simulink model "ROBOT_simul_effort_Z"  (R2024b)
settings: Solver=VariableStepAuto  StartTime=0.0  StopTime=5  RelTol=1e-3
undefined symbols (not defined in the file): a, ARRIERE_Defaut_sldprt, avant01_Defaut_sldprt, avant02_Defaut_sldprt, avant03_Defaut_sldprt, avant1_Defaut_sldprt, AXE, BASE_Defaut_sldprt, BIELLE, BIELLE_Defaut_sldprt, BRAS_Defaut_sldprt, bras_Defaut_sldprt, C_Realiste_sldprt, CABLE_Defaut_sldprt, cable_Defaut_sldprt, CACHE_Defaut_sldprt, CARTE, carte_Defaut_sldprt, CARTER, carter, CHC, CODEUR_Defaut_sldprt, cruciforme, cylindrique, deg, Drive, Fichiers, Fichiers_Matlab_sujetA, FIXATION, fixation_Defaut_sldprt, H, HEXAGONALE_Defaut_sldprt, joint_Defaut_sldprt, kg, m, M4, M4_Defaut_sldprt, manette1_Defaut_sldprt, manette2_Defaut_sldprt, MATLAB, Matlab, matlab_Defaut_sldprt, mm, modif, MOTEUR_Defaut_sldprt, N, NEZ_Defaut_sldprt, nom, palier, PARALLELOGRAMME_Defaut_sldprt, petite, plaque, rad, Ressort, Rondelle, ROTOR_Defaut_sldprt, s, SET, simple, socle_Defaut_sldprt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
libraries: sm_lib x463, fl_lib x45, nesl_utility x27, simulink x2
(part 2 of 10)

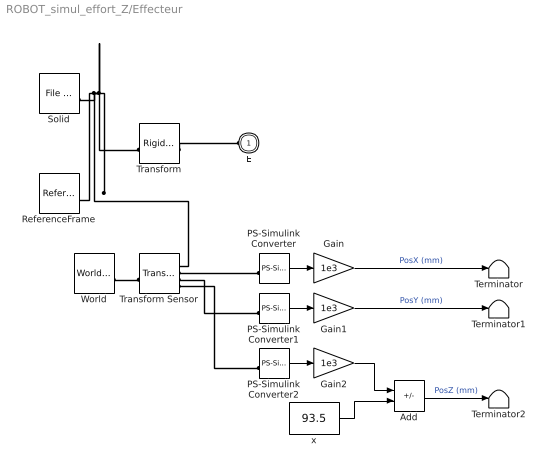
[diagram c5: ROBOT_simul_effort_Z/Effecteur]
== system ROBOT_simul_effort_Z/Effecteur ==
  Add : Sum  Inputs=+-
  Gain : Gain  Gain=1e3
  Gain1 : Gain  Gain=1e3
  Gain2 : Gain  Gain=1e3
  PS-Simulink Converter : nesl_utility/PS-Simulink Converter  PhysicalDomain=network_engine_domain  SubClassName=ps_output  LeftPortType=input  RightPortType=output  PseudoPeriodic=off  Frequencies=[]  VectorFormat=1-D array  Unit=1  AffineConversion=off
  PS-Simulink Converter1 : nesl_utility/PS-Simulink Converter  PhysicalDomain=network_engine_domain  SubClassName=ps_output  LeftPortType=input  RightPortType=output  PseudoPeriodic=off  Frequencies=[]  VectorFormat=1-D array  Unit=1  AffineConversion=off
  PS-Simulink Converter2 : nesl_utility/PS-Simulink Converter  PhysicalDomain=network_engine_domain  SubClassName=ps_output  LeftPortType=input  RightPortType=output  PseudoPeriodic=off  Frequencies=[]  VectorFormat=1-D array  Unit=1  AffineConversion=off
  ReferenceFrame : sm_lib/Frames and Transforms/Reference Frame
  Solid : sm_lib/Body Elements/File Solid  ExtGeomFileName=/MATLAB Drive/Fichiers_Matlab_sujetA/Fichiers Matlab/STL/manette2_Defaut_sldprt.STL  UnitType=Custom  ExtGeomFileUnits=mm  StepReaderType=HEX  ExportConvexHullGeometry=off  InertiaType=Custom  BasedOnType=Density  Density=1000  DensityUnits=kg/(m^3)  Mass=0.053  MassUnits=kg  CenterOfMass=[0 0 35.7]  CenterOfMassUnits=mm  MomentsOfInertia=[11.53195593564609 11.464562757624146 11.477456236480506]  MomentsOfInertiaUnits=kg*mm^2  ProductsOfInertia=[-0.014032469477280249 0.0038968914795150661 0.025527028661124163]  ProductsOfInertiaUnits=kg*mm^2  GraphicType=FromGeometry  MarkerShape=Sphere  MarkerSize=10  GraphicVisPropType=SimpleVisualProperties  GraphicDiffuseColor=[1 1 1]  GraphicOpacity=1  GraphicSpecularColor=[0.5 0.5 0.5 1.0]  GraphicAmbientColor=[0.15 0.15 0.15 1.0]  GraphicEmissiveColor=[0.0 0.0 0.0 1.0]  GraphicShininess=75  DoExposeReferenceFrame=on  SerializedFrames=<Frames/>
  Terminator : Terminator
  Terminator1 : Terminator
  Terminator2 : Terminator
  Transform : sm_lib/Frames and Transforms/Rigid Transform  RotationMethod=ArbitraryAxis  FollAlignAxisA=+X  BaseAlignAxisA=+Y  FollAlignAxisB=+Y  BaseAlignAxisB=+Z  RotationStandardAxis=+Z  RotationAngle=2.2920311904365782  RotationAngleUnits=rad  RotationArbitraryAxis=[0.63063758405056181 -0.45231899713116352 0.63063758405056158]  RotationSequenceAxes=FollowerAxes  RotationSequence=XYX  RotationSequenceAngles=[0 0 0]  RotationSequenceAnglesUnits=deg  RotationMatrix=[1 0 0; 0 1 0; 0 0 1]  Quaternion=[1 0 0 0]  TranslationMethod=Cartesian  TranslationCartesianOffset=[-0.52204305767083048 1.5422448888264837 -2.2456176397956377e-14]  TranslationCartesianOffsetUnits=mm  TranslationStandardAxis=+Z  TranslationStandardOffset=0  TranslationStandardOffsetUnits=mm  TranslationROffset=0  TranslationROffsetUnits=m  TranslationThetaOffset=0  TranslationThetaOffsetUnits=deg  TranslationZOffset=0  TranslationZOffsetUnits=m
  Transform Sensor : sm_lib/Frames and Transforms/Transform Sensor  MeasurementFrame=World  RotationSequence=XYX  SenseAngle=off  SenseAxis=off  SenseQ=off  SenseR=off  SenseRotationSequence=off  SenseOmegaX=off  SenseOmegaY=off  SenseOmegaZ=off  SenseOmega=off  SenseQDot=off  SenseRDot=off  SenseRotationSequenceDot=off  SenseAlphaX=off  SenseAlphaY=off  SenseAlphaZ=off  SenseAlpha=off  SenseQDDot=off  SenseRDDot=off  SenseX=on  SenseY=on  SenseZ=on  SenseXYZ=off  SenseRad=off  SenseAzim=off  SenseDist=off  SenseInc=off  SenseXDot=off  SenseYDot=off  SenseZDot=off  SenseXYZDot=off  SenseRadDot=off  SenseAzimDot=off  SenseDistDot=off  SenseIncDot=off  SenseXDDot=off  SenseYDDot=off  SenseZDDot=off  SenseXYZDDot=off  SenseRadDDot=off  SenseAzimDDot=off  SenseDistDDot=off  SenseIncDDot=off
  World : sm_lib/Frames and Transforms/World Frame
  x : Constant  Value=93.5
  E : PMIOPort  Side=Left
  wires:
  Gain1/1 -> Terminator1/1  "PosY (mm)"
  PS-Simulink Converter2/1 -> Gain2/1
  x/1 -> Add/2
  Add/1 -> Terminator2/1  "PosZ (mm)"
  PS-Simulink Converter1/1 -> Gain1/1
  Gain2/1 -> Add/1
  PS-Simulink Converter/1 -> Gain/1
  Gain/1 -> Terminator/1  "PosX (mm)"
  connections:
  Solid/RConn1 -- ReferenceFrame/RConn1 -- Transform Sensor/RConn1 -- Transform/LConn1
  Transform/RConn1 -- E/RConn1
  Transform Sensor/RConn3 -- PS-Simulink Converter1/LConn1
  World/RConn1 -- Transform Sensor/LConn1
  PS-Simulink Converter2/LConn1 -- Transform Sensor/RConn4
  Transform Sensor/RConn2 -- PS-Simulink Converter/LConn1

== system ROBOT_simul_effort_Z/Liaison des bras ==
  EFFECTEUR_1_RIGID : Subsystem
  manette_1_RIGID : Subsystem
  E1 : PMIOPort  Side=Left
  E2 : PMIOPort  Port=2  Side=Left
  S1 : PMIOPort  Port=3  Side=Right
  E3 : PMIOPort  Port=4  Side=Left
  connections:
  EFFECTEUR_1_RIGID/RConn1 -- manette_1_RIGID/LConn1
  S1/RConn1 -- manette_1_RIGID/RConn1
  EFFECTEUR_1_RIGID/LConn1 -- E2/RConn1
  EFFECTEUR_1_RIGID/LConn3 -- E1/RConn1
  EFFECTEUR_1_RIGID/LConn2 -- E3/RConn1

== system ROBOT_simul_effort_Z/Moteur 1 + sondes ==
  In1 : Inport
  Moteur courant continu1 : Subsystem
  Reference electrique : fl_lib/Electrical/Electrical Elements/Electrical Reference
  Simulink-PS Converter1 : nesl_utility/Simulink-PS Converter  PhysicalDomain=network_engine_domain  SubClassName=ps_input  LeftPortType=input  RightPortType=output  PseudoPeriodic=off  Frequencies=[]  NoiseDistribution=none  NoiseParameters=[]  Unit=V  AffineConversion=off  FilteringAndDerivatives=zero  SimscapeFilterOrder=2  InputFilterTimeConstant=1e-4  UdotUserProvided=1
  Sondes electriques1 : Subsystem
  Source de tension controlée1 : fl_lib/Electrical/Electrical Sources/Controlled Voltage Source
  Conn1 : PMIOPort  Side=Right
  Conn2 : PMIOPort  Port=2  Side=Right
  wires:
  In1/1 -> Simulink-PS Converter1/1
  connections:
  Conn2/RConn1 -- Moteur courant continu1/RConn2
  Conn1/RConn1 -- Moteur courant continu1/RConn1
  Source de tension controlée1/LConn1 -- Sondes electriques1/LConn1
  Simulink-PS Converter1/RConn1 -- Source de tension controlée1/RConn1
  Sondes electriques1/RConn2 -- Source de tension controlée1/RConn2 -- Reference electrique/LConn1 -- Moteur courant continu1/LConn2
  Sondes electriques1/RConn1 -- Moteur courant continu1/LConn1

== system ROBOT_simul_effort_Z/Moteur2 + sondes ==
  In1 : Inport
  Moteur courant continu2 : Subsystem
  Reference electrique : fl_lib/Electrical/Electrical Elements/Electrical Reference
  Simulink-PS Converter1 : nesl_utility/Simulink-PS Converter  PhysicalDomain=network_engine_domain  SubClassName=ps_input  LeftPortType=input  RightPortType=output  PseudoPeriodic=off  Frequencies=[]  NoiseDistribution=none  NoiseParameters=[]  Unit=V  AffineConversion=off  FilteringAndDerivatives=zero  SimscapeFilterOrder=2  InputFilterTimeConstant=1e-4  UdotUserProvided=1
  Sondes electriques : Subsystem
  Source de tension controlée : fl_lib/Electrical/Electrical Sources/Controlled Voltage Source
  Conn1 : PMIOPort  Side=Right
  Conn2 : PMIOPort  Port=2  Side=Right
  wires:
  In1/1 -> Simulink-PS Converter1/1
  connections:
  Sondes electriques/RConn1 -- Moteur courant continu2/LConn1
  Source de tension controlée/RConn2 -- Reference electrique/LConn1 -- Sondes electriques/RConn2 -- Moteur courant continu2/LConn2
  Simulink-PS Converter1/RConn1 -- Source de tension controlée/RConn1
  Source de tension controlée/LConn1 -- Sondes electriques/LConn1
  Conn1/RConn1 -- Moteur courant continu2/RConn1
  Conn2/RConn1 -- Moteur courant continu2/RConn2

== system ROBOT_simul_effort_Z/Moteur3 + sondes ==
  In1 : Inport
  Moteur courant continu3 : Subsystem
  Reference electrique : fl_lib/Electrical/Electrical Elements/Electrical Reference
  Simulink-PS Converter1 : nesl_utility/Simulink-PS Converter  PhysicalDomain=network_engine_domain  SubClassName=ps_input  LeftPortType=input  RightPortType=output  PseudoPeriodic=off  Frequencies=[]  NoiseDistribution=none  NoiseParameters=[]  Unit=V  AffineConversion=off  FilteringAndDerivatives=zero  SimscapeFilterOrder=2  InputFilterTimeConstant=1e-4  UdotUserProvided=1
  Sondes electriques3 : Subsystem
  Source de tension controlée3 : fl_lib/Electrical/Electrical Sources/Controlled Voltage Source
  Conn1 : PMIOPort  Side=Right
  Conn2 : PMIOPort  Port=2  Side=Right
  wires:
  In1/1 -> Simulink-PS Converter1/1
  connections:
  Sondes electriques3/RConn1 -- Moteur courant continu3/LConn1
  Moteur courant continu3/LConn2 -- Reference electrique/LConn1 -- Source de tension controlée3/RConn2 -- Sondes electriques3/RConn2
  Simulink-PS Converter1/RConn1 -- Source de tension controlée3/RConn1
  Source de tension controlée3/LConn1 -- Sondes electriques3/LConn1
  Conn1/RConn1 -- Moteur courant continu3/RConn1
  Conn2/RConn1 -- Moteur courant continu3/RConn2

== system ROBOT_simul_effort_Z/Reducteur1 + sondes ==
  Conv en tr/s : Gain  Gain=-60/(2*pi)
  Conv w : nesl_utility/PS-Simulink Converter  PhysicalDomain=network_engine_domain  SubClassName=ps_output  LeftPortType=input  RightPortType=output  PseudoPeriodic=off  Frequencies=[]  VectorFormat=1-D array  Unit=1  AffineConversion=off
  Conv w1 : nesl_utility/PS-Simulink Converter  PhysicalDomain=network_engine_domain  SubClassName=ps_output  LeftPortType=input  RightPortType=output  PseudoPeriodic=off  Frequencies=[]  VectorFormat=1-D array  Unit=1  AffineConversion=off
  Invers signe : Gain  Gain=-1
  Reference mecanique : fl_lib/Mechanical/Rotational Elements/Mechanical Rotational Reference
  Rotational Hard Stop : fl_lib/Mechanical/Rotational Elements/Rotational Hard Stop  Commented=on  upper_bnd=0 rad  lower_bnd=-1.95 rad  model=simscape.enum.hardstop.fulldamped  stiff_up=1e+4 N*m/rad  stiff_low=1e+4 N*m/rad  D_up=100 N*m/(rad/s)  D_low=100 N*m/(rad/s)  transition=0.001 rad  coeff_rest=0.7  w_tol=0.1 rad/s  trq_tol=0.001 N*m  w_specify=off  w_priority=None  w=0 rad/s  w_nominal_specify=off  w_nominal_value=1  w_nominal_unit=rad/s  t_specify=off  t_priority=None  t=0 N*m  t_nominal_specify=off  t_nominal_value=1  t_nominal_unit=N*m  phi_specify=on  phi_priority=High  phi=0 rad  phi_nominal_specify=off  phi_nominal_value=1  phi_nominal_unit=rad  M_specify=off  M_priority=None  M=0
  Réducteur de vitesse : fl_lib/Mechanical/Mechanisms/Gear Box  ratio=-7.627  t_in_specify=off  t_in_priority=None  t_in=0 N*m  t_in_nominal_specify=off  t_in_nominal_value=1  t_in_nominal_unit=N*m  t_out_specify=off  t_out_priority=None  t_out=0 N*m  t_out_nominal_specify=off  t_out_nominal_value=1  t_out_nominal_unit=N*m
  Sonde omega /theta1 : fl_lib/Mechanical/Mechanical Sensors/Ideal Rotational Motion Sensor  reference=foundation.enum.MeasurementReference.difference  acceleration_port=false  velocity_port=true  position_port=true  wrap_angle=false  offset=0 rad
  Terminator : Terminator
  Terminator1 : Terminator
  E1 : PMIOPort  Side=Left
  Ref : PMIOPort  Port=2  Side=Left
  S1 : PMIOPort  Port=3  Side=Right
  Ref1 : PMIOPort  Port=4  Side=Right
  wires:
  Conv w1/1 -> Invers signe/1  "Angle_mot1 (rad)"
  Invers signe/1 -> Terminator1/1  "Angle_mot1 (rad)"
  Conv w/1 -> Conv en tr/s/1
  Conv en tr/s/1 -> Terminator/1  "Nmoteur1 (tr/min)"
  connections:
  Sonde omega /theta1/LConn1 -- E1/RConn1 -- Réducteur de vitesse/LConn1
  Reference mecanique/LConn1 -- Ref/RConn1 -- Ref1/RConn1 -- Rotational Hard Stop/RConn1 -- Sonde omega /theta1/RConn1
  Conv w/LConn1 -- Sonde omega /theta1/RConn2
  Conv w1/LConn1 -- Sonde omega /theta1/RConn3
  Réducteur de vitesse/RConn1 -- Rotational Hard Stop/LConn1 -- S1/RConn1

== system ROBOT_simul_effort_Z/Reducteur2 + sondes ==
  Conv en tr/s : Gain  Gain=60/(2*pi)
  Conv en ° : Gain  Gain=180/pi
  Conv w : nesl_utility/PS-Simulink Converter  PhysicalDomain=network_engine_domain  SubClassName=ps_output  LeftPortType=input  RightPortType=output  PseudoPeriodic=off  Frequencies=[]  VectorFormat=1-D array  Unit=1  AffineConversion=off
  Conv w1 : nesl_utility/PS-Simulink Converter  PhysicalDomain=network_engine_domain  SubClassName=ps_output  LeftPortType=input  RightPortType=output  PseudoPeriodic=off  Frequencies=[]  VectorFormat=1-D array  Unit=1  AffineConversion=off
  Reference mecanique : fl_lib/Mechanical/Rotational Elements/Mechanical Rotational Reference
  Rotational Hard Stop : fl_lib/Mechanical/Rotational Elements/Rotational Hard Stop  Commented=on  upper_bnd=1.95 rad  lower_bnd=0 rad  model=simscape.enum.hardstop.fulldamped  stiff_up=1e+4 N*m/rad  stiff_low=1e+4 N*m/rad  D_up=100 N*m/(rad/s)  D_low=100 N*m/(rad/s)  transition=0.001 rad  coeff_rest=0.7  w_tol=0.1 rad/s  trq_tol=0.001 N*m  w_specify=off  w_priority=None  w=0 rad/s  w_nominal_specify=off  w_nominal_value=1  w_nominal_unit=rad/s  t_specify=off  t_priority=None  t=0 N*m  t_nominal_specify=off  t_nominal_value=1  t_nominal_unit=N*m  phi_specify=on  phi_priority=High  phi=0 rad  phi_nominal_specify=off  phi_nominal_value=1  phi_nominal_unit=rad  M_specify=off  M_priority=None  M=0
  Réducteur de vitesse2 : fl_lib/Mechanical/Mechanisms/Gear Box  ratio=7.627  t_in_specify=off  t_in_priority=None  t_in=0 N*m  t_in_nominal_specify=off  t_in_nominal_value=1  t_in_nominal_unit=N*m  t_out_specify=off  t_out_priority=None  t_out=0 N*m  t_out_nominal_specify=off  t_out_nominal_value=1  t_out_nominal_unit=N*m
  Sonde omega /theta2 : fl_lib/Mechanical/Mechanical Sensors/Ideal Rotational Motion Sensor  reference=foundation.enum.MeasurementReference.difference  acceleration_port=false  velocity_port=true  position_port=true  wrap_angle=false  offset=0 rad
  Terminator : Terminator
  Terminator1 : Terminator
  E1 : PMIOPort  Side=Left
  Ref : PMIOPort  Port=2  Side=Left
  S1 : PMIOPort  Port=3  Side=Right
  Ref1 : PMIOPort  Port=4  Side=Right
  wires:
  Conv w1/1 -> Conv en °/1  "Angle_mot2 (rad)"
  Conv en °/1 -> Terminator1/1  "Angle_mot2 (°)"
  Conv w/1 -> Conv en tr/s/1
  Conv en tr/s/1 -> Terminator/1  "Nmoteur2 (tr/min)"
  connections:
  Sonde omega /theta2/LConn1 -- E1/RConn1 -- Réducteur de vitesse2/LConn1
  Ref1/RConn1 -- Sonde omega /theta2/RConn1 -- Reference mecanique/LConn1 -- Ref/RConn1 -- Rotational Hard Stop/RConn1
  Conv w1/LConn1 -- Sonde omega /theta2/RConn3
  Conv w/LConn1 -- Sonde omega /theta2/RConn2
  Réducteur de vitesse2/RConn1 -- Rotational Hard Stop/LConn1 -- S1/RConn1

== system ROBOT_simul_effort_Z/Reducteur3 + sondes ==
  Conv en tr/s : Gain  Gain=60/(2*pi)
  Conv en ° : Gain  Gain=180/pi
  Conv w : nesl_utility/PS-Simulink Converter  PhysicalDomain=network_engine_domain  SubClassName=ps_output  LeftPortType=input  RightPortType=output  PseudoPeriodic=off  Frequencies=[]  VectorFormat=1-D array  Unit=1  AffineConversion=off
  Conv w1 : nesl_utility/PS-Simulink Converter  PhysicalDomain=network_engine_domain  SubClassName=ps_output  LeftPortType=input  RightPortType=output  PseudoPeriodic=off  Frequencies=[]  VectorFormat=1-D array  Unit=1  AffineConversion=off
  Reference mecanique : fl_lib/Mechanical/Rotational Elements/Mechanical Rotational Reference
  Rotational Hard Stop : fl_lib/Mechanical/Rotational Elements/Rotational Hard Stop  Commented=on  upper_bnd=1.95 rad  lower_bnd=0 rad  model=simscape.enum.hardstop.fulldamped  stiff_up=1e+4 N*m/rad  stiff_low=1e+4 N*m/rad  D_up=100 N*m/(rad/s)  D_low=100 N*m/(rad/s)  transition=0.001 rad  coeff_rest=0.7  w_tol=0.1 rad/s  trq_tol=0.001 N*m  w_specify=off  w_priority=None  w=0 rad/s  w_nominal_specify=off  w_nominal_value=1  w_nominal_unit=rad/s  t_specify=off  t_priority=None  t=0 N*m  t_nominal_specify=off  t_nominal_value=1  t_nominal_unit=N*m  phi_specify=on  phi_priority=High  phi=0 rad  phi_nominal_specify=off  phi_nominal_value=1  phi_nominal_unit=rad  M_specify=off  M_priority=None  M=0
  Réducteur de vitesse3 : fl_lib/Mechanical/Mechanisms/Gear Box  ratio=7.627  t_in_specify=off  t_in_priority=None  t_in=0 N*m  t_in_nominal_specify=off  t_in_nominal_value=1  t_in_nominal_unit=N*m  t_out_specify=off  t_out_priority=None  t_out=0 N*m  t_out_nominal_specify=off  t_out_nominal_value=1  t_out_nominal_unit=N*m
  Sonde omega /theta2 : fl_lib/Mechanical/Mechanical Sensors/Ideal Rotational Motion Sensor  reference=foundation.enum.MeasurementReference.difference  acceleration_port=false  velocity_port=true  position_port=true  wrap_angle=false  offset=0 rad
  Terminator : Terminator
  Terminator1 : Terminator
  E1 : PMIOPort  Side=Left
  Ref : PMIOPort  Port=2  Side=Left
  S1 : PMIOPort  Port=3  Side=Right
  Ref1 : PMIOPort  Port=4  Side=Right
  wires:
  Conv w1/1 -> Conv en °/1  "Angle_mot3 (rad)"
  Conv en °/1 -> Terminator1/1  "Angle_mot3 (°)"
  Conv w/1 -> Conv en tr/s/1
  Conv en tr/s/1 -> Terminator/1  "Nmoteur3 (tr/min)"
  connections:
  Sonde omega /theta2/LConn1 -- E1/RConn1 -- Réducteur de vitesse3/LConn1
  Ref/RConn1 -- Reference mecanique/LConn1 -- Rotational Hard Stop/RConn1 -- Ref1/RConn1 -- Sonde omega /theta2/RConn1
  Conv w1/LConn1 -- Sonde omega /theta2/RConn3
  Réducteur de vitesse3/RConn1 -- Rotational Hard Stop/LConn1 -- S1/RConn1
  Conv w/LConn1 -- Sonde omega /theta2/RConn2

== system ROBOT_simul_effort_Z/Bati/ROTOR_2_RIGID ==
  CODEUR_1_RIGID : Subsystem
  ROTOR_1_RIGID : Subsystem
  ReferenceFrame : sm_lib/Frames and Transforms/Reference Frame
  Transform : sm_lib/Frames and Transforms/Rigid Transform  RotationMethod=ArbitraryAxis  FollAlignAxisA=+X  BaseAlignAxisA=+Y  FollAlignAxisB=+Y  BaseAlignAxisB=+Z  RotationStandardAxis=+Z  RotationAngle=2.0943951023931953  RotationAngleUnits=rad  RotationArbitraryAxis=[0.57735026918962584 0.57735026918962562 0.57735026918962584]  RotationSequenceAxes=FollowerAxes  RotationSequence=XYX  RotationSequenceAngles=[0 0 0]  RotationSequenceAnglesUnits=deg  RotationMatrix=[1 0 0; 0 1 0; 0 0 1]  Quaternion=[1 0 0 0]  TranslationMethod=Cartesian  TranslationCartesianOffset=[30.900000000000009 0 -2.4868995751603507e-14]  TranslationCartesianOffsetUnits=mm  TranslationStandardAxis=+Z  TranslationStandardOffset=0  TranslationStandardOffsetUnits=mm  TranslationROffset=0  TranslationROffsetUnits=m  TranslationThetaOffset=0  TranslationThetaOffsetUnits=deg  TranslationZOffset=0  TranslationZOffsetUnits=m
  Transform1 : sm_lib/Frames and Transforms/Rigid Transform  RotationMethod=ArbitraryAxis  FollAlignAxisA=+X  BaseAlignAxisA=+Y  FollAlignAxisB=+Y  BaseAlignAxisB=+Z  RotationStandardAxis=+Z  RotationAngle=1.9381695666920589  RotationAngleUnits=rad  RotationArbitraryAxis=[0.51405666735189148 -0.51405666735189148 0.68665237602598705]  RotationSequenceAxes=FollowerAxes  RotationSequence=XYX  RotationSequenceAngles=[0 0 0]  RotationSequenceAnglesUnits=deg  RotationMatrix=[1 0 0; 0 1 0; 0 0 1]  Quaternion=[1 0 0 0]  TranslationMethod=Cartesian  TranslationCartesianOffset=[30.899999999999991 0 0]  TranslationCartesianOffsetUnits=mm  TranslationStandardAxis=+Z  TranslationStandardOffset=0  TranslationStandardOffsetUnits=mm  TranslationROffset=0  TranslationROffsetUnits=m  TranslationThetaOffset=0  TranslationThetaOffsetUnits=deg  TranslationZOffset=0  TranslationZOffsetUnits=m
  Transform2 : sm_lib/Frames and Transforms/Rigid Transform  RotationMethod=ArbitraryAxis  FollAlignAxisA=+X  BaseAlignAxisA=+Y  FollAlignAxisB=+Y  BaseAlignAxisB=+Z  RotationStandardAxis=+Z  RotationAngle=1.624664356272121  RotationAngleUnits=rad  RotationArbitraryAxis=[-0.22603347840136132 0.22603347840136129 0.94753244444903439]  RotationSequenceAxes=FollowerAxes  RotationSequence=XYX  RotationSequenceAngles=[0 0 0]  RotationSequenceAnglesUnits=deg  RotationMatrix=[1 0 0; 0 1 0; 0 0 1]  Quaternion=[1 0 0 0]  TranslationMethod=Cartesian  TranslationCartesianOffset=[-36.399999999999999 0 0]  TranslationCartesianOffsetUnits=mm  TranslationStandardAxis=+Z  TranslationStandardOffset=0  TranslationStandardOffsetUnits=mm  TranslationROffset=0  TranslationROffsetUnits=m  TranslationThetaOffset=0  TranslationThetaOffsetUnits=deg  TranslationZOffset=0  TranslationZOffsetUnits=m
  F : PMIOPort  Side=Left
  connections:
  ReferenceFrame/RConn1 -- Transform/LConn1 -- Transform1/LConn1 -- Transform2/LConn1
  Transform/RConn1 -- F/RConn1
  ROTOR_1_RIGID/LConn1 -- Transform1/RConn1
  CODEUR_1_RIGID/LConn1 -- Transform2/RConn1

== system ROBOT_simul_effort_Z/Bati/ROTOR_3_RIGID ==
  CODEUR_1_RIGID : Subsystem
  ROTOR_1_RIGID : Subsystem
  ReferenceFrame : sm_lib/Frames and Transforms/Reference Frame
  Transform : sm_lib/Frames and Transforms/Rigid Transform  RotationMethod=ArbitraryAxis  FollAlignAxisA=+X  BaseAlignAxisA=+Y  FollAlignAxisB=+Y  BaseAlignAxisB=+Z  RotationStandardAxis=+Z  RotationAngle=2.0943951023931953  RotationAngleUnits=rad  RotationArbitraryAxis=[0.57735026918962562 0.57735026918962584 0.57735026918962595]  RotationSequenceAxes=FollowerAxes  RotationSequence=XYX  RotationSequenceAngles=[0 0 0]  RotationSequenceAnglesUnits=deg  RotationMatrix=[1 0 0; 0 1 0; 0 0 1]  Quaternion=[1 0 0 0]  TranslationMethod=Cartesian  TranslationCartesianOffset=[30.899999999999984 -7.1054273576010019e-15 1.7763568394002505e-15]  TranslationCartesianOffsetUnits=mm  TranslationStandardAxis=+Z  TranslationStandardOffset=0  TranslationStandardOffsetUnits=mm  TranslationROffset=0  TranslationROffsetUnits=m  TranslationThetaOffset=0  TranslationThetaOffsetUnits=deg  TranslationZOffset=0  TranslationZOffsetUnits=m
  Transform1 : sm_lib/Frames and Transforms/Rigid Transform  RotationMethod=ArbitraryAxis  FollAlignAxisA=+X  BaseAlignAxisA=+Y  FollAlignAxisB=+Y  BaseAlignAxisB=+Z  RotationStandardAxis=+Z  RotationAngle=1.9381695666920589  RotationAngleUnits=rad  RotationArbitraryAxis=[0.51405666735189148 -0.51405666735189148 0.68665237602598705]  RotationSequenceAxes=FollowerAxes  RotationSequence=XYX  RotationSequenceAngles=[0 0 0]  RotationSequenceAnglesUnits=deg  RotationMatrix=[1 0 0; 0 1 0; 0 0 1]  Quaternion=[1 0 0 0]  TranslationMethod=Cartesian  TranslationCartesianOffset=[30.899999999999999 0 0]  TranslationCartesianOffsetUnits=mm  TranslationStandardAxis=+Z  TranslationStandardOffset=0  TranslationStandardOffsetUnits=mm  TranslationROffset=0  TranslationROffsetUnits=m  TranslationThetaOffset=0  TranslationThetaOffsetUnits=deg  TranslationZOffset=0  TranslationZOffsetUnits=m
  Transform2 : sm_lib/Frames and Transforms/Rigid Transform  RotationMethod=ArbitraryAxis  FollAlignAxisA=+X  BaseAlignAxisA=+Y  FollAlignAxisB=+Y  BaseAlignAxisB=+Z  RotationStandardAxis=+Z  RotationAngle=1.624664356272121  RotationAngleUnits=rad  RotationArbitraryAxis=[-0.22603347840136134 0.22603347840136132 0.94753244444903439]  RotationSequenceAxes=FollowerAxes  RotationSequence=XYX  RotationSequenceAngles=[0 0 0]  RotationSequenceAnglesUnits=deg  RotationMatrix=[1 0 0; 0 1 0; 0 0 1]  Quaternion=[1 0 0 0]  TranslationMethod=Cartesian  TranslationCartesianOffset=[-36.399999999999999 0 0]  TranslationCartesianOffsetUnits=mm  TranslationStandardAxis=+Z  TranslationStandardOffset=0  TranslationStandardOffsetUnits=mm  TranslationROffset=0  TranslationROffsetUnits=m  TranslationThetaOffset=0  TranslationThetaOffsetUnits=deg  TranslationZOffset=0  TranslationZOffsetUnits=m
  F : PMIOPort  Side=Left
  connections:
  Transform/LConn1 -- ReferenceFrame/RConn1 -- Transform1/LConn1 -- Transform2/LConn1
  Transform/RConn1 -- F/RConn1
  ROTOR_1_RIGID/LConn1 -- Transform1/RConn1
  CODEUR_1_RIGID/LConn1 -- Transform2/RConn1
